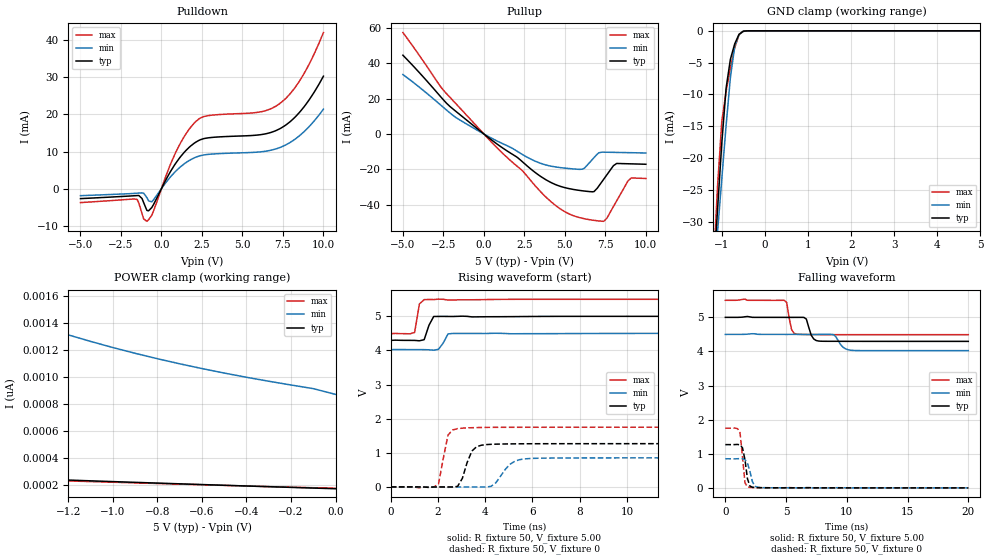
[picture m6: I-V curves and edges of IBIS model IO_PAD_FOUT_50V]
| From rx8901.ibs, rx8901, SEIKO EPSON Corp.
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[Model]   IO_PAD_FOUT_50V
Model_type 3-state
Enable Active-High
Polarity Non-Inverting
Vmeas=2.50
C_comp   2.5p   2.0p   3.0p
[Temperature Range] 25   105   -40
[Voltage Range]   5.00   4.50   5.50
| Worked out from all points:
|   slope of the pulldown table from 0 to 0.75 V, typ, clamps not added: 126 ohm
|   slope of the pullup table from 0 to 0.75 V, typ, clamps not added: 143 ohm
|   GND clamp passes 1 mA (typ) near -0.63 V on its own axis
|   falling waveform, R_fixture 50, V_fixture 5.00: 20-80 % time 403ps typ, 565ps min, 312ps max; typ from 5 V to 4.29 V
|   falling waveform, R_fixture 50, V_fixture 0: 20-80 % time 329ps typ, 388ps min, 290ps max; typ from 1.27 V to 0 V
|   rising waveform, R_fixture 50, V_fixture 5.00: 20-80 % time 239ps typ, 250ps min, 147ps max; typ from 4.29 V to 5 V
|   rising waveform, R_fixture 50, V_fixture 0: 20-80 % time 380ps typ, 590ps min, 296ps max; typ from 0 V to 1.27 V
[Pullup]
-5V       44.6mA     33.65mA    57.43mA
-2.4V     18.33mA    14.29mA    23.76mA
-900mV    6.649mA    4.756mA    8.977mA
2.9V      -19.85mA   -14.22mA   -26.45mA
3.9V      -26.28mA   -17.71mA   -36.32mA
5V        -30.37mA   -19.32mA   -44mA
6.1V      -32.18mA   -19.89mA   -47.77mA
6.8V      -32.6mA    -13.36mA   -48.89mA
7.4V      -25.59mA   -10.29mA   -49.43mA
8.2V      -16.68mA   -10.43mA   -37.84mA
8.9V      -16.85mA   -10.55mA   -26.5mA
10V       -17.13mA   -10.75mA   -25.19mA
[Pulldown]
-5V       -2.695mA   -1.898mA   -3.76mA
-1.5V     -1.871mA   -1.232mA   -2.909mA
-1.1V     -3.756mA   -1.223mA   -8.145mA
-900mV    -5.868mA   -2.416mA   -8.805mA
-600mV    -5.116mA   -3.564mA   -7.202mA
900mV     6.952mA    4.772mA    9.936mA
2V        12.16mA    8.239mA    17.55mA
2.7V      13.56mA    9.131mA    19.52mA
6.1V      14.53mA    9.907mA    20.68mA
7.3V      16.12mA    11.06mA    22.91mA
8.6V      20.95mA    14.55mA    29.52mA
10V       30.3mA     21.42mA    42.06mA
[GND Clamp]
-5V       -506.4mA   -413.2mA   -621.4mA
-1.2V     -38.91mA   -40.17mA   -37.89mA
-1.1V     -28.19mA   -31.69mA   -24.51mA
-1V       -17.6mA    -23.23mA   -14.19mA
-900mV    -8.974mA   -14.82mA   -9.506mA
-800mV    -4.446mA   -7.293mA   -5.815mA
-700mV    -2.032mA   -2.409mA   -2.638mA
-600mV    -545.5uA   -567.8uA   -606uA
-500mV    -57.02uA   -91.22uA   -35.65uA
5V        171.8pA    1.03nA     153.2pA
[POWER Clamp]
-5V       543.1pA    7.361nA    417.9pA
-4.3V     467.3pA    5.372nA    379.1pA
-3.5V     394.4pA    3.691nA    340pA
-1.7V     266pA      1.607nA    253.6pA
-1.6V     259.9pA    1.541nA    248.8pA
-1.4V     247.9pA    1.42nA     239.2pA
-1.2V     236.3pA    1.314nA    229.7pA
-900mV    219.3pA    1.177nA    215.5pA
-600mV    202.9pA    1.064nA    201.3pA
-400mV    192.3pA    999.1pA    192.1pA
-100mV    176.9pA    914.7pA    179.3pA
0V        171.8pA    871.9pA    175.5pA
[Falling Waveform]
R_fixture=50
V_fixture=5.00
V_fixture_min=4.50
V_fixture_max=5.50
0s        5V         4.5V       5.5V
4.848ns   4.999V     4.5V       5.5V
5.051ns   4.999V     4.5V       5.433V
5.455ns   4.999V     4.5V       4.64V
5.859ns   4.999V     4.5V       4.509V
6.667ns   4.951V     4.499V     4.495V
7.071ns   4.476V     4.499V     4.494V
7.677ns   4.305V     4.499V     4.493V
10.3ns    4.297V     4.036V     4.492V
20ns      4.295V     4.024V     4.492V
[Falling Waveform]
R_fixture=50
V_fixture=0
V_fixture_min=0
V_fixture_max=0
0s        1.268V     852.2mV    1.75V
1.01ns    1.274V     853.8mV    1.735V
1.212ns   1.259V     858.3mV    1.609V
1.414ns   1.172V     856.7mV    908.1mV
1.616ns   823.9mV    828.4mV    147.4mV
1.818ns   271.1mV    729.6mV    33.89mV
2.02ns    53.95mV    487.5mV    14.26mV
2.424ns   9.976mV    48.72mV    7.183mV
2.828ns   4.934mV    10.66mV    5.364mV
20ns      66.33uV    58.87uV    91.86uV
[Rising Waveform]
R_fixture=50
V_fixture=5.00
V_fixture_min=4.50
V_fixture_max=5.50
0s        4.295V     4.024V     4.492V
1.01ns    4.294V     4.024V     4.529V
1.212ns   4.283V     4.024V     5.362V
1.414ns   4.316V     4.024V     5.491V
1.616ns   4.737V     4.018V     5.493V
1.818ns   4.997V     4.008V     5.492V
2.02ns    4.997V     4.034V     5.504V
2.424ns   4.997V     4.484V     5.476V
2.626ns   4.995V     4.499V     5.48V
20ns      5V         4.5V       5.5V
[Rising Waveform]
R_fixture=50
V_fixture=0
V_fixture_min=0
V_fixture_max=0
0s        3.447nV    5.992nV    3.272nV
2.02ns    -112uV     -1.968mV   82mV
2.424ns   -937.9uV   -11.72mV   1.522V
2.828ns   15.83mV    -128.4uV   1.709V
3.434ns   1.052V     -54.31uV   1.736V
4.04ns    1.241V     -1.953mV   1.745V
4.444ns   1.253V     117.3mV    1.747V
5.051ns   1.261V     664.8mV    1.748V
5.859ns   1.265V     831.4mV    1.749V
20ns      1.268V     852.2mV    1.75V
[Ramp]
R_load=50
dV/dt_r   7.608E-1/3.651E-10   5.113E-1/5.748E-10   1.050E+0/2.492E-10
dV/dt_f   4.228E-1/3.728E-10   2.856E-1/5.577E-10   6.048E-1/2.647E-10
|[End   IO_PAD_FOUT_50V
